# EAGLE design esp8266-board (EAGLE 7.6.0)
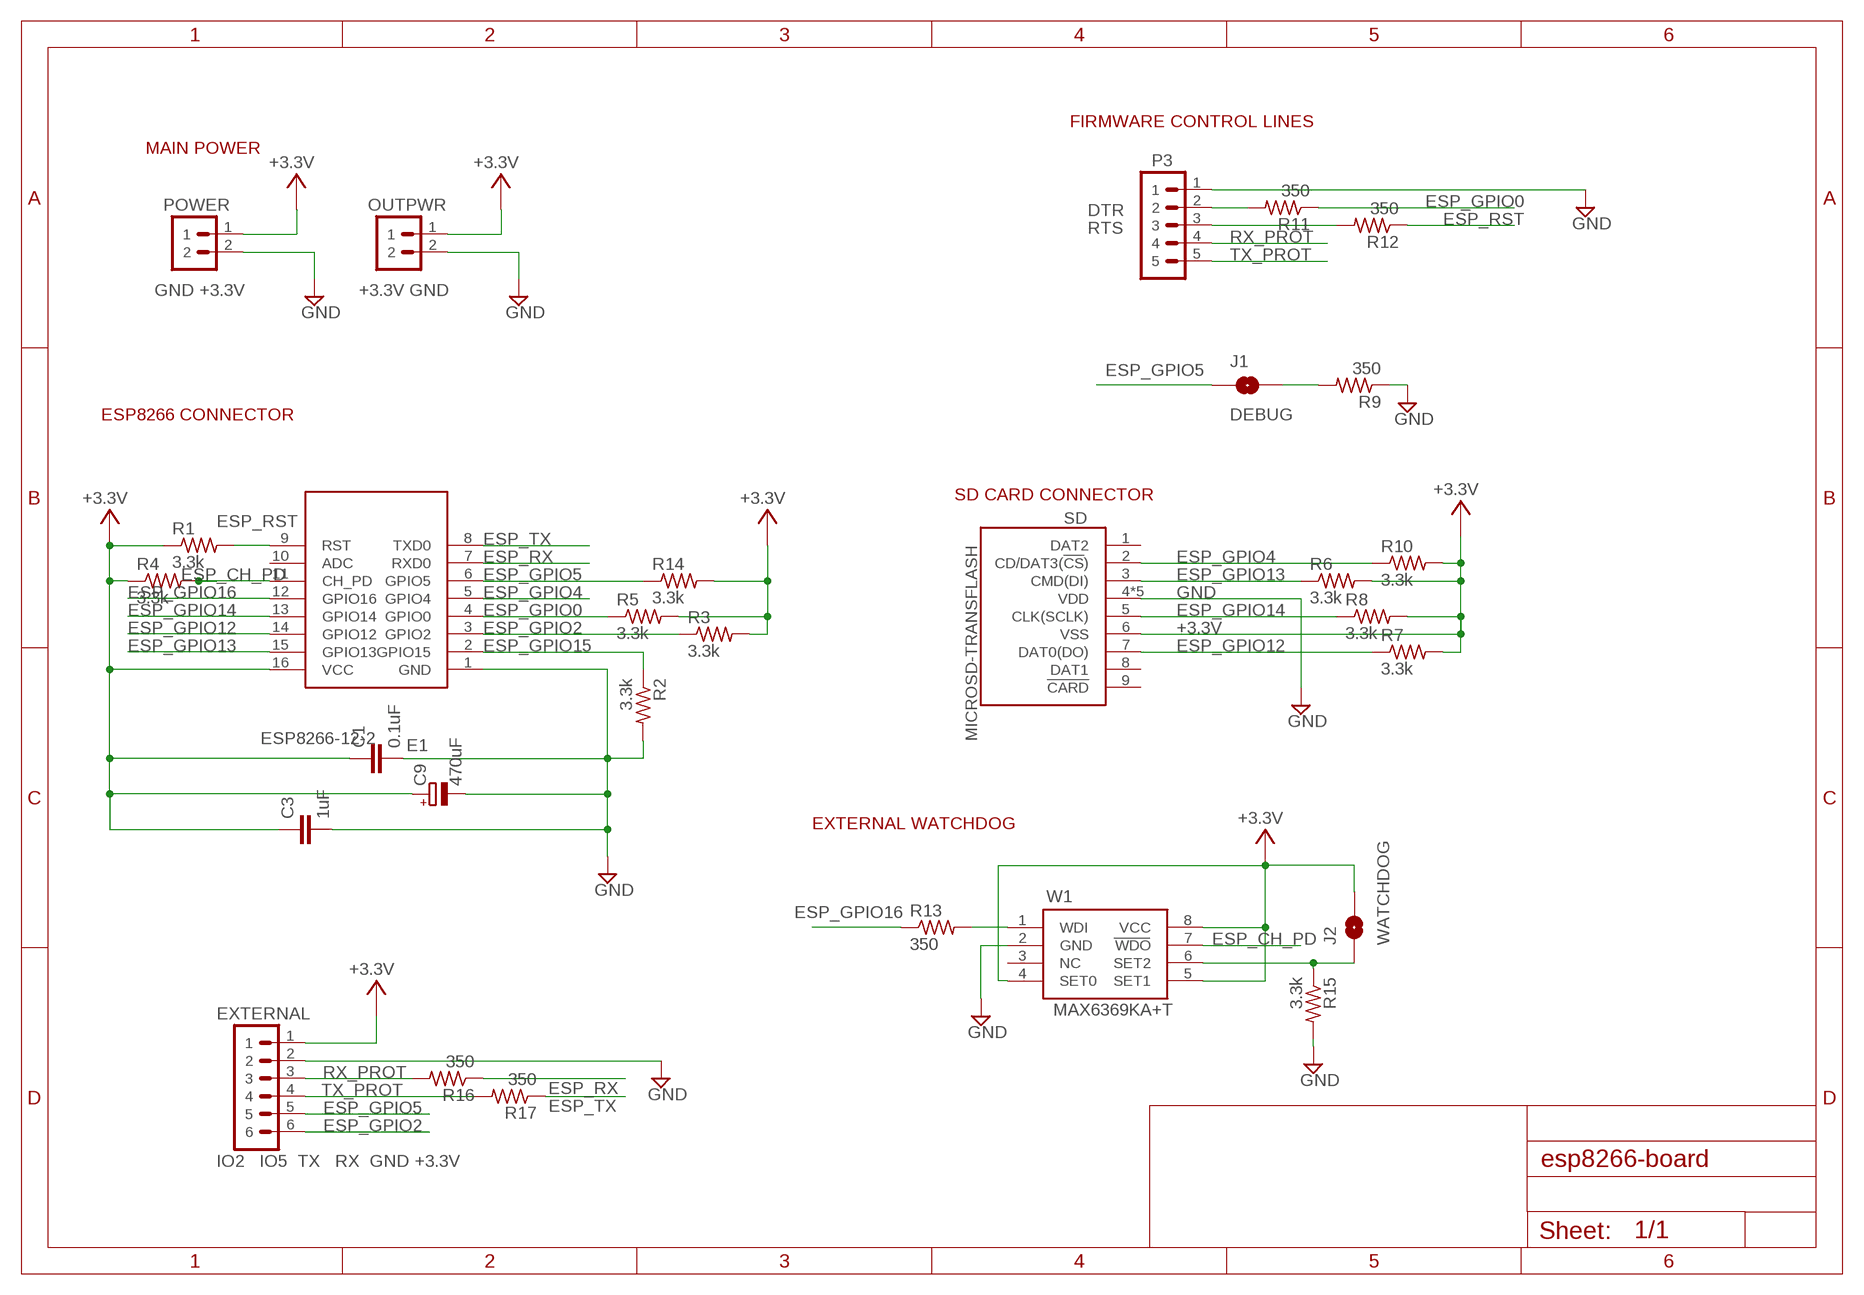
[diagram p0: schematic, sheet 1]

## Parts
C1  0.1uF  CAPACITOR0805  [SMD0805@1]
C3  1uF  CAPACITOR0805  [SMD0805@1]
C9  470uF  CPOL-EUE2.5-6  [E2,5-6]
E1  ESP8266-12-2  [ESP8266-12-2]
EXTERNAL  IO2 IO5 TX RX GND +3.3V  PIN-HEADER-6PIN  [PIN-HEADER-6PIN]
J1  DEBUG  JUMPER-PAD-2ROUND  [JUMPER-PAD-2-ROUND]
J2  WATCHDOG  JUMPER-PAD-2ROUND  [JUMPER-PAD-2-ROUND]
OUTPWR  +3.3V GND  PIN-HEADER-2PIN  [PIN-HEADER-2PIN]
P3  GND DTR RTS RX TX  PIN-HEADER-5PIN  [PIN-HEADER-5PIN]
POWER  GND +3.3V  PIN-HEADER-2PIN  [PIN-HEADER-2PIN]
R1  3.3k  RESISTOR0805  [SMD0805]
R2  3.3k  RESISTOR0805  [SMD0805]
R3  3.3k  RESISTOR0805  [SMD0805]
R4  3.3k  RESISTOR0805  [SMD0805]
R5  3.3k  RESISTOR0805  [SMD0805]
R6  3.3k  RESISTOR0805  [SMD0805]
R7  3.3k  RESISTOR0805  [SMD0805]
R8  3.3k  RESISTOR0805  [SMD0805]
R9  350  RESISTOR0805  [SMD0805]
R10  3.3k  RESISTOR0805  [SMD0805]
R11  350  RESISTOR0805  [SMD0805]
R12  350  RESISTOR0805  [SMD0805]
R13  350  RESISTOR0805  [SMD0805]
R14  3.3k  RESISTOR0805  [SMD0805]
R15  3.3k  RESISTOR0805  [SMD0805]
R16  350  RESISTOR0805  [SMD0805]
R17  350  RESISTOR0805  [SMD0805]
SD  MICROSD-TRANSFLASH  [MICROSD-TRANSFLASH]
W1  MAX6369KA+T  MAX6369-74  [SOT23-8]

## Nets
+3.3V [power-1A]: C1.1 C3.1 C9.+ E1.16(VCC) EXTERNAL.1 J2.2 OUTPWR.1 POWER.1 R1.1 R3.2 R4.1 R5.2 R6.2 R7.2 R8.2 R10.2 R14.2 SD.6(VSS) W1.4(SET0) W1.5(SET1) W1.8(VCC)
ESP_CH_PD: E1.11(CH_PD) R4.2 W1.7(WDO)
ESP_GPIO0: E1.4(GPIO0) R5.1 R11.1
ESP_GPIO2: E1.3(GPIO2) EXTERNAL.6 R3.1
ESP_GPIO4: E1.5(GPIO4) R10.1 SD.2(CD/DAT3(!CS!))
ESP_GPIO5: E1.6(GPIO5) EXTERNAL.5 J1.1 R14.1
ESP_GPIO12: E1.14(GPIO12) R7.1 SD.7(DAT0(DO))
ESP_GPIO13: E1.15(GPIO13) R6.1 SD.3(CMD(DI))
ESP_GPIO14: E1.13(GPIO14) R8.1 SD.5(CLK(SCLK))
ESP_GPIO15: E1.2(GPIO15) R2.1
ESP_GPIO16: E1.12(GPIO16) R13.1
ESP_RST: E1.9(RST) R1.2 R12.1
ESP_RX: E1.7(RXD0) R16.1
ESP_TX: E1.8(TXD0) R17.1
GND [power-1A]: C1.2 C3.2 C9.- E1.1(GND) EXTERNAL.2 OUTPWR.2 P3.1 POWER.2 R2.2 R9.1 R15.2 SD.4(VDD) SD.S1(VDD) SD.S2(VDD) SD.S3(VDD) SD.S4(VDD) W1.2(GND)
N$1: J2.1 R15.1 W1.6(SET2)
N$6: J1.2 R9.2
N$7: P3.2 R11.2
N$8: P3.3 R12.2
N$10: R13.2 W1.1(WDI)
RX_PROT: EXTERNAL.3 P3.4 R16.2
TX_PROT: EXTERNAL.4 P3.5 R17.2
Unconnected: E1.10(ADC) SD.1(DAT2) SD.8(DAT1) SD.9(!CARD) W1.3(NC)

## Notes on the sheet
- FIRMWARE CONTROL LINES
- MAIN POWER
- DTR
- RTS
- ESP8266 CONNECTOR
- SD CARD CONNECTOR
- EXTERNAL WATCHDOG

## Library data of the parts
C1 C3 = stutz-components-library:CAPACITOR
C9 = rcl:CPOL-EU: POLARIZED CAPACITOR, European symbol
E1 = stutz-components-library:ESP8266-12-2
EXTERNAL = stutz-components-library:PIN-HEADER-6PIN
J1 J2 = stutz-components-library:JUMPER-PAD-2
OUTPWR POWER = stutz-components-library:PIN-HEADER-2PIN
P3 = stutz-components-library:PIN-HEADER-5PIN
R1-R17 = stutz-components-library:RESISTOR
SD = stutz-components-library:MICROSD-TRANSFLASH
W1 = stutz-components-library:MAX6369-74

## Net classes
0 default: width 0.254 mm, clearance 0.16 mm
1 power-4A: width 2 mm, clearance 0.2 mm
2 comm-rs485: width 1 mm, clearance 0.2 mm
3 power-2A: width 1 mm, clearance 0.2 mm
4 power-1.7A: width 0.8 mm, clearance 0.2 mm
5 power-1A: width 0.254 mm, clearance 0.2 mm

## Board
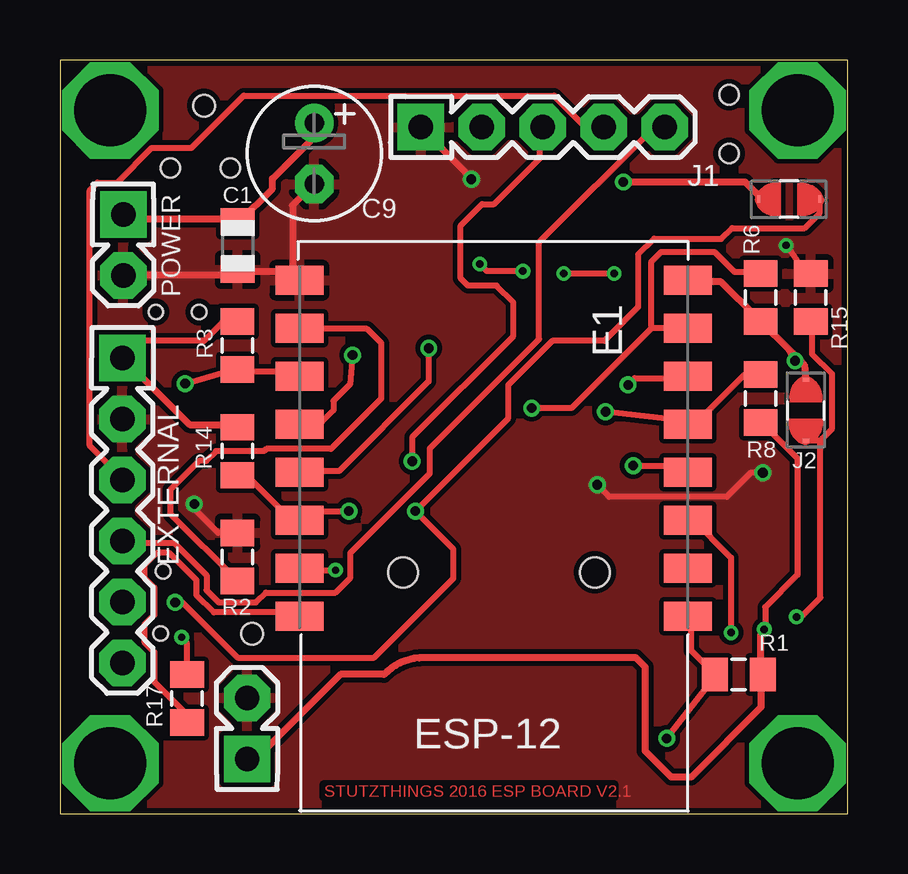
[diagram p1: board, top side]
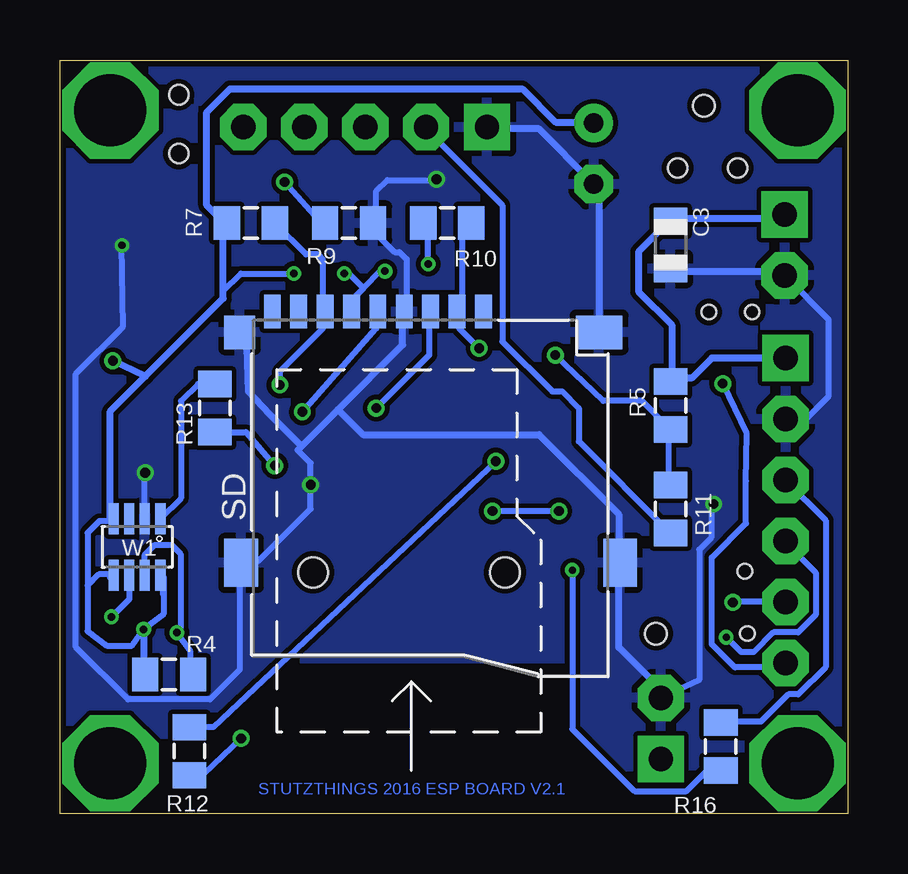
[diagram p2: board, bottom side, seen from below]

Size 32.85 x 31.4 mm. Coordinates in mm from the lower left corner, seen from the top.
Outline: 0,0 32.85,0 32.85,31.4 0,31.4 0,0
Copper layers (1*16): Top 0.035mm / dielectric 1.5mm / Bottom 0.035mm
Design rules "SeeedStudio_2layer_DRU_no_angle_20140221": minimum track width 6mil, minimum drill 12mil, track to track 6mil, track to pad 6mil, pad to pad 6mil, via to via 6mil, smd to smd 0mil, copper to edge 10mil, drill to drill 10mil, minimum pad ring 10mil, minimum via ring 6mil, stop-mask expansion 2mil, vias tented up to drill 100mil, thermal gap 10mil
Holes 0.6 mm at 4.3,10.1 4.2,7.5 4,20.9 5.8,20.9
Holes 0.9 mm at 8,7.5 6,29.5
Holes 0.8 mm at 4.6,26.9 7.1,26.9 27.9,27.5 27.9,29.95
bRestrict: area 12.1,0.8 to 24.1,6.2

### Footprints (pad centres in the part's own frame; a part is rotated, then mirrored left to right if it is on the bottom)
SMD0805@1 = smd 1.1 x 1.4: 1 -1,0; 2 1,0
E2,5-6 = drill 0.813 pad 1.6: + -1.27,0 | drill 0.813 pad 1.6 octagon: - 1.27,0
ESP8266-12-2 = smd 2 x 1.2: 1 7.818,-8.922; 2 7.818,-6.922; 3 7.818,-4.922; 4 7.818,-2.922; 5 7.818,-0.922; 6 7.818,1.078; 7 7.818,3.078; 8 7.818,5.078; 9 -8.382,5.078; 10 -8.382,3.078; 11 -8.382,1.078; 12 -8.382,-0.922; 13 -8.382,-2.922; 14 -8.382,-4.922; 15 -8.382,-6.922; 16 -8.382,-8.922
PIN-HEADER-6PIN = drill 1.016 pad 1.93 square: 1 -5.08,0 | drill 1.016 pad 1.93 octagon: 2 -2.54,0; 3 0,0; 4 2.54,0; 5 5.08,0; 6 7.62,0
JUMPER-PAD-2-ROUND = smd 0.152 x 0.305: 1 -1.27,0; 2 1.27,0
PIN-HEADER-2PIN = drill 1.016 pad 1.93 square: 1 -1.27,0 | drill 1.016 pad 1.93 octagon: 2 1.27,0
PIN-HEADER-5PIN = drill 1.016 pad 1.93 square: 1 -5.08,0 | drill 1.016 pad 1.93 octagon: 2 -2.54,0; 3 0,0; 4 2.54,0; 5 5.08,0
SMD0805 = smd 1.1 x 1.4: 1 -1,0; 2 1,0
MICROSD-TRANSFLASH = smd 1.4 x 0.7: 1 15.22,5.2; 2 15.22,6.3; 3 15.22,7.4; 4 15.22,8.5; 5 15.22,9.6; 6 15.22,10.7; 7 15.22,11.8; 8 15.22,12.9; 9 15.22,14 | smd 2 x 1.4: S1 4.75,-0.5; S2 4.75,15.3 | smd 1.4 x 1.28: S3 14.35,15.36 | smd 1.4 x 1.95: S4 14.35,0.375 | hole 1.25: 4.35,4.3; 4.35,12.3
SOT23-8 = smd 0.42 x 1.3: 1 0.936,1.08; 2 0.286,1.08; 3 -0.364,1.08; 4 -1.014,1.08; 5 -1.014,-1.27; 6 -0.364,-1.27; 7 0.286,-1.27; 8 0.936,-1.27

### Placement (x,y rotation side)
C1  7.41,23.66 270 top
C3  7.4,23.7 270 bottom
C9  10.6,27.5 270 top
E1  17.8,13.3 180 top
EXTERNAL  2.6,13.9 270 top
J1  30.4,25.6 180 top
J2  31.1,16.8 90 top
OUTPWR  7.8,3.55 90 top
P3  20.13,28.6 0 top
POWER  2.64,23.69 270 top
R1  28.3,5.8 180 top
R2  7.4,10.7 90 top
R3  7.4,19.5 90 top
R4  28.3,5.8 0 bottom
R5  7.4,17 90 bottom
R6  29.2,21.5 270 top
R7  24.9,24.6 180 bottom
R8  29.2,17.3 270 top
R9  20.8,24.6 180 bottom
R10  16.7,24.6 180 bottom
R11  7.4,12.7 270 bottom
R12  27.45,2.6 90 bottom
R13  26.4,16.9 90 bottom
R14  7.4,15.1 90 top
R15  31.3,21.5 90 top
R16  5.3,2.8 90 bottom
R17  5.3,4.8 90 top
SD  10,5.7 90 bottom
W1  29.6,11.2 0 bottom

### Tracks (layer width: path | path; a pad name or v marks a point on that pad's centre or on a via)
+3.3V  (via drill 0.31, 0.4)
  Top 0.254: R3.2 6.8,20.5 6,19.7 3.32,19.7 EXTERNAL.1 | 29.22,16.2 29.34,16.2 30.75,14.8 30.75,9.95 29.4,8.6 29.4,7.72 v29.36,7.68 | v19.3,22.6 17.8,22.6 v17.5,22.9 | v23.1,22.5 v21,22.5
  Top 0.3: R14.2 7.34,16.2 5.4,16.2 2.63,18.97 EXTERNAL.1 | POWER.1 2.77,24.93 2.91,24.79 7.34,24.79 C1.1 7.48,24.65 8.86,26.04 8.86,26.45 10.53,28.12 10.53,28.67 C9.+ | 30.4,19.32 29.22,20.5 R6.2 29.09,20.64 27.56,22.16 26.32,22.16 E1.16 | 30.4,19.32 31.02,18.7 J2.2 | v30.65,18.87 30.4,19.32 | 29.22,16.2 R8.2 | 7.2,2.08 OUTPWR.1 8.03,2.13 11.7,5.8 13.5,5.8 arc-45 15.19,6.5 24,6.5 24.4,6.1 24.4,2.61 25.48,1.52 26.32,1.52 29.22,4.43 29.22,5.68 R4.1 29.22,5.82 29.22,7.48 v29.36,7.68
  Bottom 0.254: 30.75,12.19 31.21,12.19 31.7,11.7 31.7,9.5 | 31.7,9.5 31.7,7.6 30.9,7 29.84,7 v29.36,7.68 28.53,8.31 28.53,9.14 | 30.75,9.97 31.23,9.97 31.7,9.5 | v19.3,22.6 19.4,22.7 19.4,22.6 19.5,22.6 20.2,21.9 | v17.5,22.9 17.5,24.4 R10.2 | 20.2,21.9 20.6,21.5 20.6,21.02 SD.6 | 26.04,21.47 26.04,21.76 25.3,22.5 v23.1,22.5 | v21,22.5 20.8,22.5 20.2,21.9
  Bottom 0.3: 7.48,18 R5.2 | R5.2 7.34,18.14 6.51,18.14 5.68,18.97 2.63,18.97 EXTERNAL.1 | POWER.1 2.77,24.93 2.91,24.79 7.34,24.79 C3.1 7.48,24.65 8.73,23.41 8.73,21.74 7.34,20.36 7.34,18.28 R5.2 | 28.53,9.14 28.53,9.83 W1.8 | 30.75,9.83 W1.5 30.75,9.97 | 30.75,12.19 W1.4 30.75,12.33 30.75,16.76 29.29,18.21 | v29.36,7.68 29.36,5.82 R4.1 | 29.29,18.21 26.04,21.47 26.04,24.52 R7.2 26.04,24.65 26.73,25.35 26.73,29.22 25.76,30.19 13.57,30.19 12.19,28.81 10.66,28.81 C9.+ | 29.29,18.21 v30.65,18.87
ESP_CH_PD  (via drill 0.31)
  Top 0.254: v27.98,7.54 27.98,10.66 26.32,12.33 E1.11
  Bottom 0.254: R4.2 27.42,5.82 27.42,6.79 v27.98,7.54 27.82,7.7 27.82,10.82 28.2,11.2 28.9,11.2 29.31,10.79 W1.7
ESP_GPIO0  (via drill 0.4)
  Top 0.254: v12.2,19.1 12.1,17.9 11.4,17.2 11.4,16.8 10.5,15.9 10.3,15.9 E1.4
  Bottom 0.254: 7.48,13.71 R11.1 7.48,13.78 7.48,15.93 | 7.48,15.93 R5.1 | 7.48,15.93 7.48,16.08 8.6,17.2 10.2,17.2 v12.2,19.1
ESP_GPIO2  (via drill 0.4)
  Top 0.254: E1.3 9.97,18.28 9.83,18.42 7.48,18.42 R3.1 7.34,18.42 6.92,18.42 v5.22,17.91
  Bottom 0.254: v5.22,17.91 4.22,15.82 4.25,13.85 4.25,12.1 5.68,10.66 5.68,7.06 4.71,6.09 2.77,6.09 2.63,6.23 EXTERNAL.6
ESP_GPIO4  (via drill 0.4)
  Top 0.254: v15.37,19.39 15.37,18 11.63,14.27 10.11,14.27 E1.5
  Bottom 0.254: R10.1 16.07,24.1 16.07,21.19 16.2,21.05 SD.2 16.2,20.91 16.2,20.22 v15.37,19.39
ESP_GPIO5  (via drill 0.4)
  Top 0.254: 27.56,23.96 24.76,23.96 24.1,23.3 24.1,21.1 22.7,19.7 20.53,19.7 18.7,17.87 18.7,16.48 v14.82,12.6 16.4,11.02 16.4,9.8 13.1,6.5 7.4,6.5 5.1,8.8 v4.8,8.8 | v12.05,12.6 10.39,12.6 10.11,12.33 E1.6 9.97,12.33 9.56,12.33 7.89,13.99 7.48,13.99 R14.1
  Top 0.256: 27.56,23.96 27.57,23.95 28.02,24.4 31.05,24.4 31.67,25.02 J1.1
  Bottom 0.254: v12.05,12.6 v14.82,12.6 | EXTERNAL.5 4.68,8.82 v4.8,8.8
ESP_GPIO12  (via drill 0.4)
  Top 0.254: v23.68,17.87 23.96,18.14 26.18,18.14 E1.14
  Bottom 0.254: 23.82,24.24 23.82,24.52 R7.1 22.6,23.3 22.1,23.3 21.88,23.08 21.88,21.05 SD.7 21.88,20.91 21.88,20.22 23.68,18.42 v23.68,17.87
ESP_GPIO13  (via drill 0.4)
  Top 0.254: v19.67,16.9 21.33,16.9 24.65,20.22 | 24.65,20.22 E1.15 | 24.65,20.22 24.65,22.99 25.07,23.41 27.29,23.41 28.12,22.58 29.09,22.58 R6.1
  Bottom 0.254: v19.67,16.9 17.45,19.11 17.45,20.91 SD.3
ESP_GPIO14  (via drill 0.4)
  Top 0.254: R8.1 29.09,18.28 28.53,18.28 26.59,16.34 26.32,16.34 E1.13 26.18,16.34 v22.75,16.74
  Bottom 0.254: v22.75,16.74 19.67,20.22 19.67,20.91 SD.5
ESP_GPIO15
  Top 0.254: R2.1 4.6,12.5 4.6,13.5 5.8,14.7 6.1,14.7 6.5,15.1 8.5,15.1 8.6,15.2 11.3,15.2 13.4,17.3 13.4,19.6 12.8,20.2 10,20.2 E1.2
ESP_GPIO16  (via drill 0.4)
  Top 0.254: v23.9,14.5 25.7,14.5 E1.12
  Bottom 0.254: R13.1 25.1,15.9 v23.9,14.5
ESP_RST  (via drill 0.4)
  Top 0.254: v25.3,3.13 25.4,3.29 27.29,5.68 R1.2 27.29,5.82 26.32,6.79 26.32,8.17 E1.9
  Bottom 0.254: v25.3,3.13 26.87,1.66 27.29,1.66 R12.1
ESP_RX  (via drill 0.3)
  Top 0.254: v11.49,10.14 10.04,10.14 E1.7
  Bottom 0.254: v11.49,10.14 11.49,3.52 8.9,0.93 6.73,0.93 5.9,1.76 5.38,1.76 R16.1
ESP_TX
  Top 0.254: R17.1 5.28,3.83 5.28,4.14 3.93,5.49 3.93,6.73 3.52,7.14 3.52,7.87 3.93,8.28 3.93,9.42 3.52,9.83 3.52,10.35 4.04,10.87 4.55,10.87 5.69,9.73 5.69,9.11 6.42,8.38 9.83,8.38 9.94,8.28 E1.8
GND  (via drill 0.3, 0.4)
  Top 0.254: 2.64,16.4 EXTERNAL.2 | R2.2 6.6,11.7 5.6,12.7 v5.6,12.9 | v29.3,14.2 28.8,14.2 27.8,13.2 22.9,13.2 v22.4,13.7 | v30.27,23.68 31.08,22.53 31.26,22.46 R15.2
  Top 0.3: v17.15,26.43 16.9,26.73 15.1,28.53 P3.1 | C9.- 10.53,26.18 9.7,25.35 9.7,22.71 E1.1 9.97,22.3 9.7,22.58 7.48,22.58 C1.2 7.48,22.44 2.77,22.44 POWER.2
  Bottom 0.254: EXTERNAL.2 1.76,16.44 0.8,17.4 0.8,20.58 POWER.2 | v5.6,12.9 5.7,12.8 5.7,11.5 6.2,11 6.2,5.57 OUTPWR.2 | W1.2 29.31,14.19 v29.3,14.2 | 22.94,15.14 22.4,14.6 v22.4,13.7 22.4,12.7 24.57,10.53 25.21,10.53 | 19.67,24.24 19.67,24.17 18.9,23.4 18.7,23.4 18.4,23.1 18.4,21.12 SD.4 | 19.67,24.52 19.67,25.93 19.2,26.4 17.18,26.4 v17.15,26.43 | v30.27,23.68 30.22,20.29 32.19,18.32 32.19,6.93 30.02,4.76 26.6,4.76 25.36,6 25.36,10.35 SD.S2
  Bottom 0.3: 7.76,22.58 7.48,22.58 C3.2 7.34,22.58 2.91,22.58 2.77,22.44 POWER.2 | 19.67,24.52 19.67,24.24 R9.1 | SD.S4 10.39,20.08 10.39,26.04 10.53,26.18 C9.- 10.66,26.32 12.88,28.53 14.96,28.53 P3.1 | OUTPWR.2 7.2,4.57 9.56,6.92 9.56,10.39 SD.S1 9.56,10.53 9.56,12.46 12.88,15.79 20.22,15.79 21.26,16.83 | 22.94,15.14 22.78,15.31 | 22.78,15.31 21.26,16.83 | 21.26,16.83 18.56,19.53 18.56,20.91 SD.4 | 25.21,10.53 SD.S2 | 22.78,15.31 24.09,16.63 24.99,17.58 25.05,19.44 25.35,19.94 SD.S3
  pour Bottom: -4.3,40.1 35.15,32.25 54.7,-0.8 -4.3,-1.2
  pour Top: -5.6,41.2 36.75,34 56.2,-2.2 -5.9,-2.5
N$1  (via drill 0.31)
  Top 0.254: v30.7,8.2 30.7,8 31.7,9 31.7,15.53 | 31.7,15.53 J2.1 | R15.1 31.36,20.49 31.36,19.15 32.19,18.32 32.19,16.04 31.77,15.63 31.7,15.53
  Bottom 0.254: W1.6 29.96,8.94 v30.7,8.2
N$2  (via drill 3)
  other vias: 30.75,2.1
N$3  (via drill 3)
  other vias: 2.1,2.1
N$4  (via drill 3)
  other vias: 2.1,29.3
N$5  (via drill 3)
  other vias: 30.75,29.3
N$6  (via drill 0.4)
  Top 0.254: 29.26,25.61 J1.2
  Top 0.3: 29.26,25.61 28.56,26.32 v23.48,26.32
  Bottom 0.254: v23.48,26.32 21.88,24.52 21.88,24.24 R9.2
N$7
  Bottom 0.254: R11.2 7.48,11.77 11.22,15.51 11.22,16.9 11.91,17.59 12.33,17.59 14.4,19.67 14.4,25.35 17.59,28.53 P3.2
N$8  (via drill 0.4)
  Top 0.254: v14.68,14.68 14.68,15.68 18.9,19.9 18.9,21.3 18.2,22 17,22 16.7,22.3 16.7,24.5 17.6,25.4 18.1,25.4 20,27.3 20,28.48 P3.3 20.08,28.53
  Bottom 0.254: v14.68,14.68 26.46,3.6 27.29,3.6 R12.2
N$10
  Bottom 0.254: R13.2 27.1,17.9 27.8,17.2 27.8,13.14 W1.1
RX_PROT
  Top 0.254: P3.4 22.67,28.67 21.84,28.67 20.6,29.91 7.66,29.91 5.49,27.74 3.83,27.74 2.38,26.29 1.55,26.29 1.24,25.98 1.24,15.32 2.59,13.97 EXTERNAL.3
  Bottom 0.254: R16.2 5.28,3.83 3.62,3.83 2.48,4.97 2.07,4.97 0.93,6.11 0.93,12.21 2.59,13.87 EXTERNAL.3
TX_PROT  (via drill 0.3)
  Top 0.254: v5.07,7.35 5.28,7.14 5.28,5.9 R17.2 | P3.5 25.15,28.57 24.74,28.57 19.98,23.8 19.98,19.77 15.42,15.21 15.42,14.18 12.11,10.87 12.11,9.83 11.49,9.21 8.59,9.21 8.18,8.8 6.62,8.8 6.11,9.31 6.11,9.94 4.76,11.28 2.69,11.28 EXTERNAL.4
  Bottom 0.254: v5.07,7.35 4.45,6.73 3.93,6.73 3.1,7.56 2.07,7.56 1.34,8.28 1.34,10.04 2.59,11.28 EXTERNAL.4

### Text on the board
Top: STUTZTHINGS 2016 ESP BOARD V2.1
Bottom: STUTZTHINGS 2016 ESP BOARD V2.1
